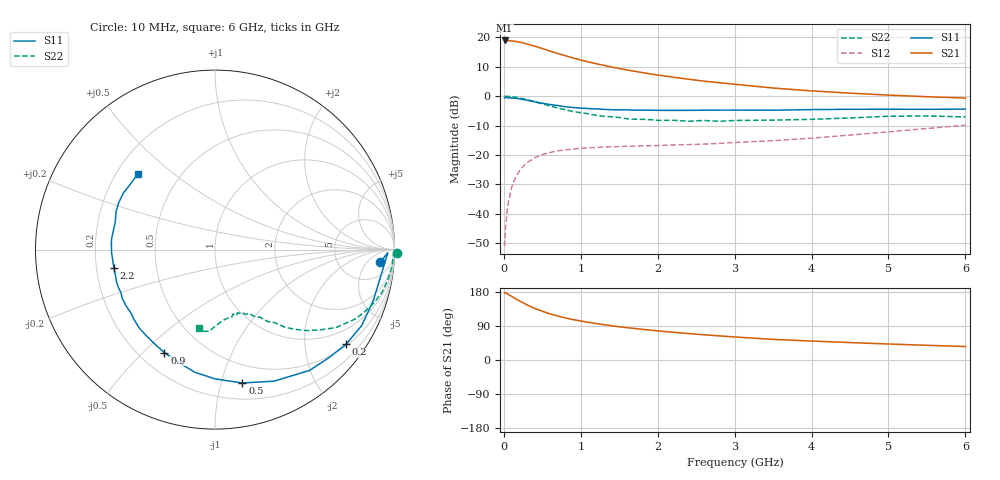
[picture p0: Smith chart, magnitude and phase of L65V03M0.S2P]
!  INFINEON TECHNOLOGIES Small Signal Semiconductors
! BFR380L3 , Si-NPN RF-Transistor in TSLP-3-1
!  Vce=5 V,  Ic=3 mA
! Common Emitter S-Parameters:  07. March 2005
#  GHz  S  MA  R  50
! f  S11  S21  S12  S22
! GHz  Mag  Ang  Mag  Ang  Mag  Ang  Mag  Ang
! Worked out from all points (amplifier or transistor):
!   36 points, 10 MHz to 6 GHz, reference 50 ohm
!   highest |S21| = 19.0 dB at 10 MHz (marker M1)
!   |S21| within 3 dB of that: start of sweep to 528 MHz
!   unconditionally stable (mu >= 1): 2.987 GHz to 4.562 GHz
!   at 250 MHz: K = 0.10, MSG = 21.0 dB, |S12| = -24.0 dB
!   at 1.4 GHz: K = 0.61, MSG = 13.6 dB, |S12| = -17.3 dB
!   at 6 GHz: K = 0.89, MSG = 4.6 dB, |S12| = -9.9 dB
!   S11 on the Smith chart (normalised r, x): 10 MHz: 13, -13; 200 MHz: 0.54, -3.01; 500 MHz: 0.33, -1.17; 900 MHz: 0.30, -0.58; 2.2 GHz: 0.27, -0.08; 6 GHz: 0.29, +0.38
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0.01  0.9242 -4.3  8.862 177.1  0.0028 81.5  1.015 -1.0
0.02  0.9632 -1.0  8.861 177.8  0.0054 92.4  0.9923 -2.0
0.05  0.935 -9.2  8.819 173.9  0.0135 84.8  0.992 -4.9
0.1  0.9265 -17.9  8.692 168.1  0.0277 80.0  0.979 -9.6
0.15  0.9204 -27.3  8.56 162.1  0.0407 75.6  0.961 -14.3
0.2  0.9009 -35.8  8.31 156.1  0.0526 72.0  0.936 -18.3
0.3  0.8547 -52.0  7.719 145.6  0.0735 63.5  0.8732 -26.2
0.4  0.8031 -65.9  7.095 136.3  0.0892 56.4  0.802 -32.8
0.5  0.7586 -78.4  6.448 128.7  0.1011 51.4  0.7374 -37.3
0.6  0.7202 -90.0  5.847 121.6  0.1102 47.0  0.6811 -41.5
0.7  0.6926 -99.3  5.32 116.2  0.1172 43.9  0.6305 -44.8
0.8  0.6607 -107.8  4.871 111.0  0.1217 41.4  0.5862 -47.8
0.9  0.6396 -116.1  4.462 106.6  0.1256 39.3  0.5465 -49.7
1.1  0.6143 -128.2  3.826 99.3  0.1323 37.2  0.4999 -53.5
1.5  0.5864 -147.7  2.96 87.7  0.1386 36.0  0.4338 -59.4
1.9  0.5775 -161.7  2.391 78.9  0.143 37.1  0.3982 -65.0
2.2  0.5722 -169.6  2.104 73.2  0.1476 39.3  0.3887 -67.1
2.6  0.5765 -178.6  1.801 66.6  0.1529 42.8  0.3856 -71.8
3.5  0.5763 164.7  1.375 54.4  0.1745 50.9  0.3911 -81.4
4.5  0.5969 154.1  1.124 46.0  0.2176 59.7  0.4254 -89.5
5.5  0.5959 142.3  0.977 38.8  0.2814 63.2  0.46 -97.6
6  0.6028 135.6  0.926 35.5  0.3205 63.0  0.4428 -101.4
